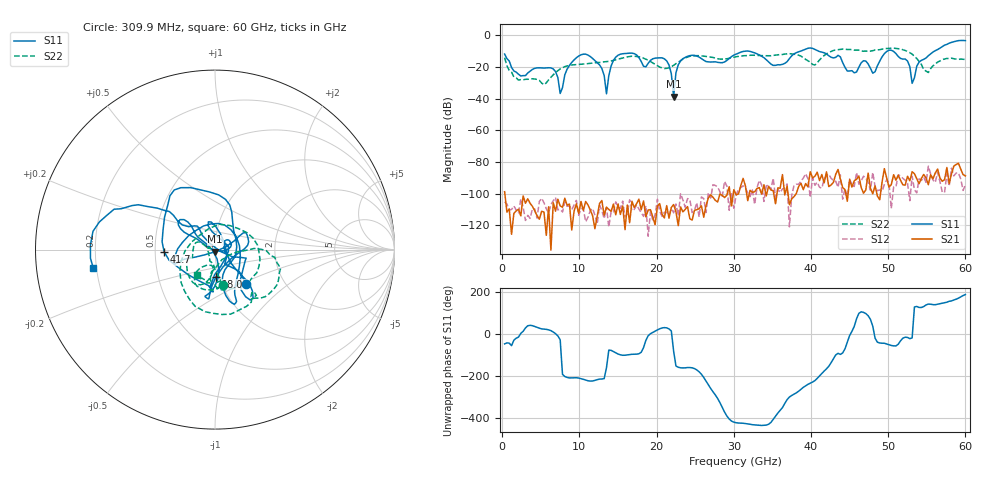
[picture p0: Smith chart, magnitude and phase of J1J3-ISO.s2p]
!Keysight Technologies,N5227A,US51270214,A.10.65.11
!Date: Thursday, October 15, 2020 08:20:34
!Correction: S11(Full 2 Port(1,2))
!S21(Full 2 Port(1,2))
!S12(Full 2 Port(1,2))
!S22(Full 2 Port(1,2))
!S2P File: Measurements: S11, S21, S12, S22:
# Hz S  dB  R 50
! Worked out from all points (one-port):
!   200 points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, 309.9 MHz to 60 GHz, reference 50 ohm
!   lowest |S11| = -38.8 dB at 22.21 GHz (marker M1), VSWR 1.02, Z = 50.1 - j1.15 ohm
!   |S11| at or under -10 dB: start of sweep to 31.36 GHz; 32.02 GHz to 38.59 GHz (6.571 GHz wide, 18.6 % of centre); 41.02 GHz to 49.85 GHz (8.827 GHz wide, 19.4 % of centre)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
!   S11 on the Smith chart (normalised r, x): 309.9 MHz: 1.30, -0.53; 18.01 GHz: 0.97, -0.30; 41.7 GHz: 0.56, -0.02; 60 GHz: 0.19, -0.07
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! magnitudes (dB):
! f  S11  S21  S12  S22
! 309.9 MHz  -11.8  -98.7  -105.2  -14.0
! 2.11 GHz  -24.5  -109.8  -112.1  -28.2
! 6.609 GHz  -21.1  -105.7  -104.5  -24.9
! 7.509 GHz  -36.7  -107.7  -109.9  -21.1
! 10.51 GHz  -11.8  -110.6  -109.5  -18.2
! 12.91 GHz  -20.9  -104.3  -110.6  -16.9
! 13.51 GHz  -36.9  -108.5  -108.5  -16.5
! 14.71 GHz  -13.7  -113.3  -105.2  -15.4
! 18.01 GHz  -16.5  -110.1  -111.9  -13.8
! 20.41 GHz  -14.1  -106.3  -111.1  -20.0
! 21.61 GHz  -18.7  -115.4  -113.5  -20.5
! 22.21 GHz  -38.8  -106.9  -112.0  -18.8
! 23.41 GHz  -14.7  -111.5  -103.9  -15.0
! 30.3 GHz  -11.8  -100.7  -100.8  -13.4
! 40.2 GHz  -8.1  -90.0  -90.0  -18.3
! 41.7 GHz  -10.9  -93.2  -90.8  -12.7
! 48 GHz  -23.8  -100.0  -86.5  -9.6
! 50.1 GHz  -9.3  -95.8  -93.2  -8.2
! 52.5 GHz  -16.1  -89.0  -93.4  -10.1
! 53.1 GHz  -30.3  -86.1  -88.9  -11.8
! 55.2 GHz  -12.8  -94.3  -82.6  -23.4
! 60 GHz  -3.3  -88.8  -94.3  -15.1
